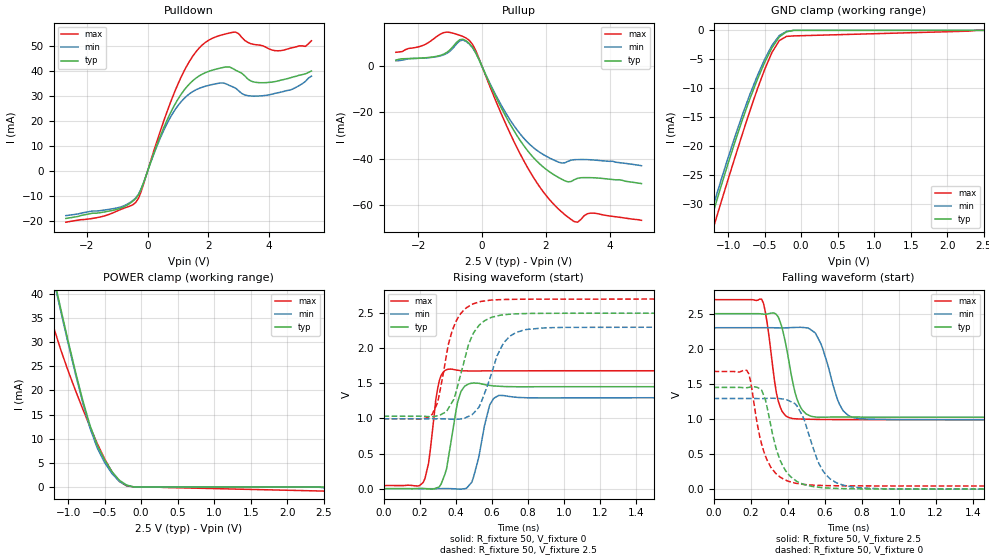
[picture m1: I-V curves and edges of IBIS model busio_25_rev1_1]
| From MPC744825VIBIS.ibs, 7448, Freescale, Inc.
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| *   60X 2.5V Model Rev1.1
[Model]   busio_25_rev1_1
Model_type   I/O
Polarity   Non-Inverting
Vinl = 0.5V
Vinh = 1.7V
Vmeas =1.25V
Cref = 0
Rref = 50
Vref = 1.25V
|   typ   min   max
C_comp   2.967499e-13   2.705084e-13   1.033671e-12
|   typ   min   max
[Voltage range]   2.5V   2.3V   2.7V
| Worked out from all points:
|   slope of the pulldown table from 0 to 0.375 V, typ, clamps not added: 29.6 ohm
|   slope of the pullup table from 0 to 0.375 V, typ, clamps not added: 32.5 ohm
|   GND clamp passes 1 mA (typ) near -0.28 V on its own axis
|   POWER clamp passes 1 mA (typ) near -0.26 V on its own axis
|   falling waveform, R_fixture 50, V_fixture 2.5: 20-80 % time 68ps typ, 89ps min, 52.8ps max; typ from 2.5 V to 1.03 V
|   rising waveform, R_fixture 50, V_fixture 0: 20-80 % time 55.6ps typ, 64.5ps min, 45.1ps max; typ from 0.001 V to 1.45 V
|   falling waveform, R_fixture 50, V_fixture 0: 20-80 % time 93.4ps typ, 109ps min, 86.3ps max; typ from 1.45 V to 0.002 V
|   rising waveform, R_fixture 50, V_fixture 2.5: 20-80 % time 101ps typ, 113ps min, 88.9ps max; typ from 1.03 V to 2.5 V
[Pulldown]
|   Voltage   I(typ)   I(min)   I(max)
-2.7V     -19.02mA   -17.9mA    -20.53mA
-1V       -15.33mA   -14.78mA   -16.01mA
-400mV    -11.14mA   -10.91mA   -12.68mA
-200mV    -6.892mA   -6.67mA    -7.709mA
400mV     13.45mA    12.73mA    15.39mA
800mV     24.4mA     22.54mA    28.94mA
1.4V      35.12mA    31.06mA    44.33mA
1.9V      39.31mA    33.88mA    51.43mA
2.9V      40.3mA     33.12mA    55.57mA
3.8V      35.3mA     30.1mA     50.06mA
4.4V      36.36mA    31.56mA    48.17mA
5.4V      40.01mA    37.95mA    52.1mA
[GND_clamp]
-2.7V     -100.8mA   -98.75mA   -103.3mA
-1.3V     -35.58mA   -34.37mA   -38.31mA
-1.2V     -31.27mA   -30.13mA   -34.04mA
-1.1V     -27.06mA   -25.99mA   -29.84mA
-900mV    -19.03mA   -18.1mA    -21.69mA
-700mV    -11.75mA   -11mA      -13.84mA
-600mV    -8.501mA   -7.845mA   -10.16mA
-400mV    -3.009mA   -2.605mA   -3.831mA
-300mV    -1.145mA   -910.9uA   -1.769mA
-200mV    -247.3uA   -170.3uA   -1.048mA
-100mV    0A         0A         -962.8uA
2.5V      0A         0A         0A
[Pullup]
-2.7V     2.675mA    2.359mA    6.047mA
-1.2V     5.234mA    4.914mA    14.56mA
-700mV    11.47mA    10.96mA    13.43mA
-500mV    11.03mA    10.78mA    12.24mA
-200mV    6.064mA    5.856mA    6.978mA
500mV     -15.1mA    -14.2mA    -17.18mA
1.1V      -30.08mA   -27.59mA   -35.33mA
1.7V      -40.84mA   -36.2mA    -50.02mA
2.3V      -47.38mA   -40.94mA   -60.51mA
2.9V      -49.13mA   -40.48mA   -67.35mA
3.4V      -48.27mA   -40.52mA   -63.64mA
5V        -50.84mA   -43.1mA    -66.74mA
[POWER_clamp]
-2.7V     151.6mA    150.2mA    124.2mA
-1.4V     57.35mA    56.74mA    43.88mA
-1.3V     50.42mA    49.85mA    38.35mA
-1.2V     43.57mA    43.03mA    33.13mA
-1.1V     36.83mA    36.31mA    28.36mA
-800mV    17.94mA    17.45mA    16.15mA
-700mV    12.71mA    12.16mA    12.44mA
-600mV    8.616mA    8.017mA    8.95mA
-400mV    3.178mA    2.773mA    3.125mA
-300mV    1.399mA    1.147mA    1.166mA
-200mV    389.9uA    287uA      221.5uA
2.5V      0A         -170.3uA   -859.2uA
|   typ   min   max
[Ramp]
dV/dt_r   0.86901/5.49274e-11   0.77480/6.42915e-11   0.97854/4.44605e-11
dV/dt_f   0.88084/6.76002e-11   0.78290/8.66960e-11   1.02306/5.26720e-11
[Falling Waveform]
R_fixture = 50
V_fixture = 2.5
V_fixture_min = 2.3
V_fixture_max = 2.7
| time   V(typ)   V(min)   V(max)
0s        2.5V       2.3V       2.7V
260ps     2.496V     2.3V       2.706V
350ps     2.453V     2.298V     1.254V
410ps     1.781V     2.301V     1.018V
450ps     1.292V     2.305V     1.002V
500ps     1.073V     2.299V     998mV
580ps     1.026V     2.074V     993.8mV
680ps     1.029V     1.214V     992.2mV
750ps     1.028V     1.026V     991.9mV
2ns       1.026V     989.3mV    991.8mV
[Rising Waveform]
R_fixture = 50
V_fixture = 0
V_fixture_min = 0
V_fixture_max = 0
| time   V(typ)   V(min)   V(max)
0s        1.42mV     589.3uV    45.81mV
220ps     3.982mV    660.3uV    88.67mV
250ps     -1.518mV   575.6uV    361.7mV
300ps     17.59mV    1.2mV      1.42V
350ps     284.7mV    2.548mV    1.695V
410ps     1.22V      -3.758mV   1.687V
480ps     1.497V     63.66mV    1.676V
590ps     1.47V      1.195V     1.677V
640ps     1.459V     1.328V     1.678V
2ns       1.452V     1.295V     1.678V
[Falling Waveform]
R_fixture = 50
V_fixture = 0
V_fixture_min = 0
V_fixture_max = 0
| time   V(typ)   V(min)   V(max)
0s        1.45V      1.292V     1.677V
180ps     1.446V     1.292V     1.692V
200ps     1.455V     1.292V     1.542V
260ps     1.41V      1.291V     641.2mV
340ps     563mV      1.294V     215.5mV
400ps     229.4mV    1.27V      118mV
480ps     76.26mV    1.051V     71.51mV
590ps     21.89mV    266.3mV    53.61mV
700ps     9.273mV    58.39mV    49.11mV
2ns       2.192mV    1.442mV    46.08mV
[Rising Waveform]
R_fixture = 50
V_fixture = 2.5
V_fixture_min = 2.3
V_fixture_max = 2.7
| time   V(typ)   V(min)   V(max)
0s        1.032V     995.1mV    994.8mV
270ps     1.026V     995.3mV    1.059V
300ps     1.038V     995.8mV    1.223V
380ps     1.229V     989.5mV    2.24V
430ps     1.641V     994.5mV    2.496V
500ps     2.219V     1.075V     2.633V
540ps     2.348V     1.216V     2.665V
660ps     2.473V     2.045V     2.692V
770ps     2.492V     2.252V     2.697V
2ns       2.499V     2.299V     2.699V
